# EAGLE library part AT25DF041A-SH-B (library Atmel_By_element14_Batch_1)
4-megabit Minimum SPI Serial Flash Memory
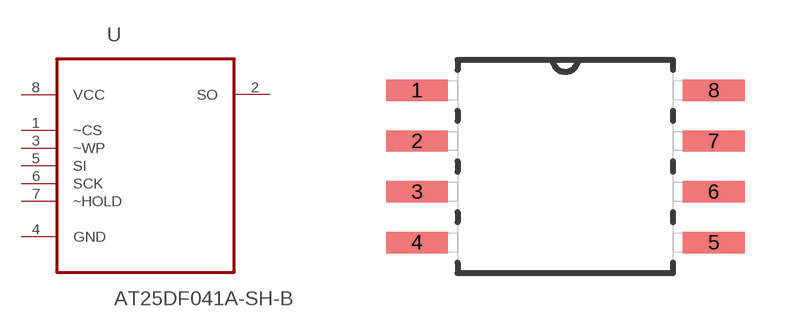
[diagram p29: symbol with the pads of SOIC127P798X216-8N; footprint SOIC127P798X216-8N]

Designator prefix U

## AT25DF041A-SH-B (MPN: AT25DF041A-SH-B; OC_FARNELL: 1715440; OC_NEWARK: 15R0305; PACKAGE: SOIC-8; SUPPLIER: Atmel)  [SOIC127P798X216-8N]
1  ~CS  in
2  SO  out
3  ~WP  in
4  GND  pas
5  SI  in
6  SCK  in
7  ~HOLD  in
8  VCC  pwr

## Footprint SOIC127P798X216-8N (pad centres in mm)
smd 1.549 x 0.533: 1 -3.708,1.905; 2 -3.708,0.635; 3 -3.708,-0.635; 4 -3.708,-1.905; 5 3.708,-1.905; 6 3.708,-0.635; 7 3.708,0.635; 8 3.708,1.905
